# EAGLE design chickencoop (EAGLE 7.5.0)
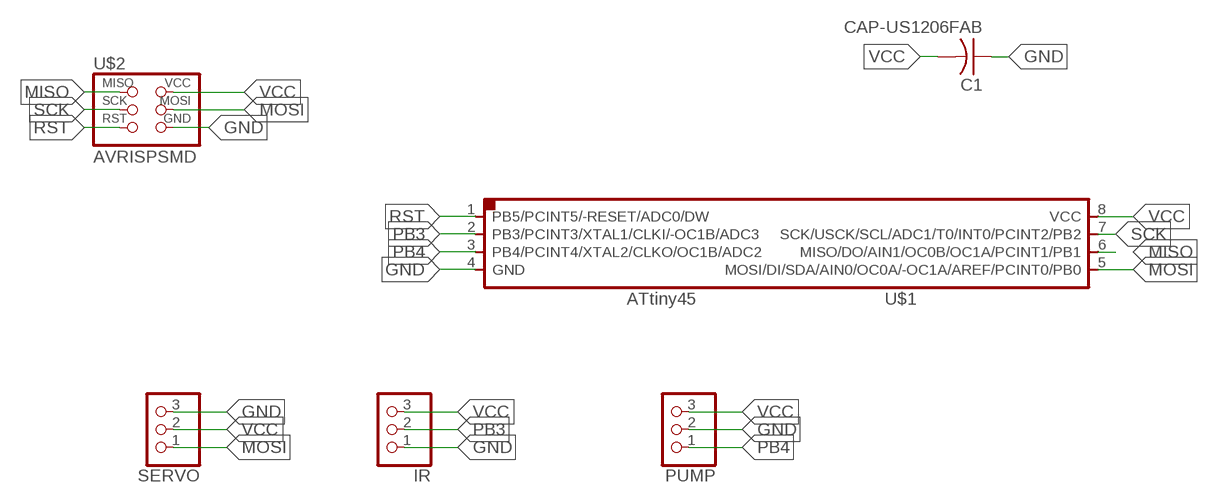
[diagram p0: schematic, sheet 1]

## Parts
C1  CAP-US1206FAB  [C1206FAB]
IR  PINHD-1X3  [1X03]
PUMP  PINHD-1X3  [1X03]
SERVO  PINHD-1X3  [1X03]
U$1  ATTINY45SI  [SOIC8]
U$2  AVRISPSMD  [2X03SMD]

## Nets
GND: C1.1 IR.1 PUMP.2 SERVO.3 U$1.4(GND) U$2.6(GND)
MISO: U$1.6(MISO/DO/AIN1/OC0B/OC1A/PCINT1/PB1) U$2.1(MISO)
MOSI: SERVO.1 U$1.5(MOSI/DI/SDA/AIN0/OC0A/-OC1A/AREF/PCINT0/PB0) U$2.4(MOSI)
PB3: IR.2 U$1.2(PB3/PCINT3/XTAL1/CLKI/-OC1B/ADC3)
PB4: PUMP.1 U$1.3(PB4/PCINT4/XTAL2/CLKO/OC1B/ADC2)
RST: U$1.1(PB5/PCINT5/-RESET/ADC0/DW) U$2.5(RST)
SCK: U$1.7(SCK/USCK/SCL/ADC1/T0/INT0/PCINT2/PB2) U$2.3(SCK)
VCC: C1.2 IR.3 PUMP.3 SERVO.2 U$1.8(VCC) U$2.2(VCC)

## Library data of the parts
C1 = fab:CAP-US
IR PUMP SERVO = pinhead:PINHD-1X3: PIN HEADER
U$1 = fab:ATTINY45
U$2 = fab:AVRISP

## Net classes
0 default: width 0.406 mm, drill 0.406 mm, clearance 0.406 mm

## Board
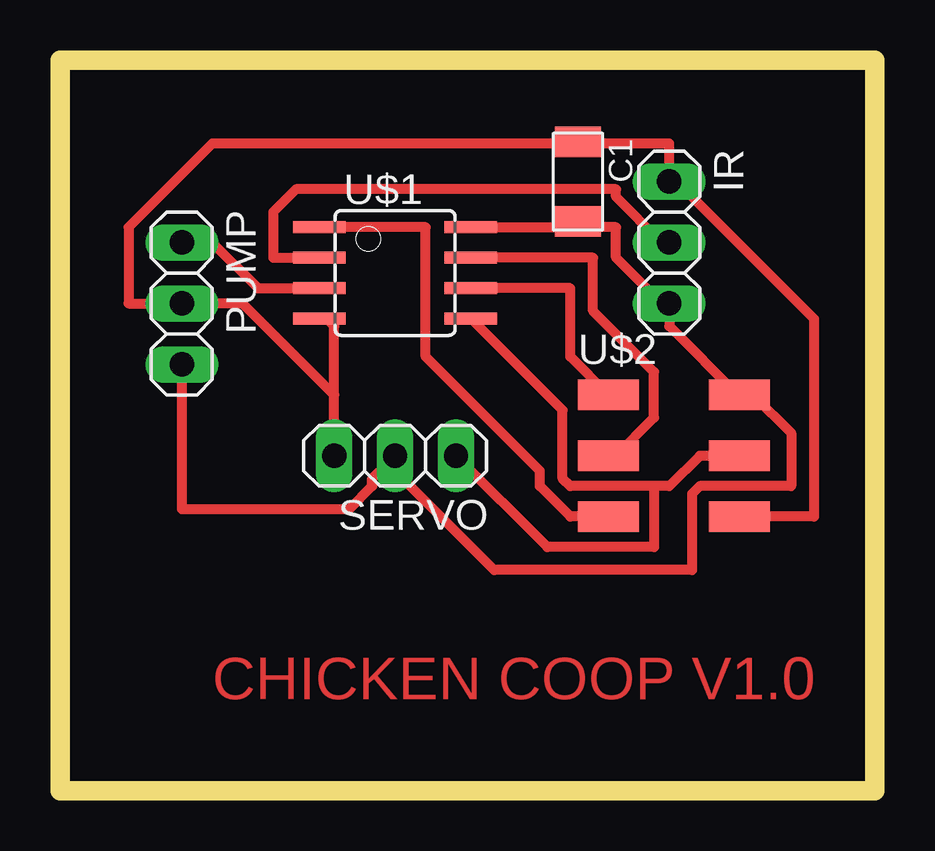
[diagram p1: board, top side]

Size 33.96 x 30.47 mm. Coordinates in mm from the lower left corner, seen from the top.
Outline: 0,0 33.96,0 33.96,30.47 0,30.47 0,0
Copper layers (1*16): Top 0.035mm / dielectric 1.5mm / Bottom 0.035mm
Design rules "default *": minimum track width 10mil, minimum drill 24mil, track to track 17mil, track to pad 17mil, pad to pad 17mil, via to via 17mil, smd to smd 8mil, copper to edge 40mil, drill to drill 8mil, minimum pad ring 10mil, minimum via ring 8mil, stop-mask expansion 4mil, vias tented up to drill 0mil, thermal gap 10mil

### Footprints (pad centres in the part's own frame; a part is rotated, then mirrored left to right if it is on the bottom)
C1206FAB = smd 1.27 x 1.905: 1 -1.651,0; 2 1.651,0
1X03 = drill 1.016 long: 1 -2.54,0; 2 0,0; 3 2.54,0
SOIC8 = smd 0.5 x 2.2: 1 -1.905,-3.154; 2 -0.645,-3.154; 3 0.625,-3.154; 4 1.895,-3.154; 5 1.905,3.154; 6 0.635,3.154; 7 -0.635,3.154; 8 -1.905,3.154
2X03SMD = smd 2.54 x 1.27: 1 -2.54,2.54; 2 2.92,2.54; 3 -2.54,0; 4 2.92,0; 5 -2.54,-2.54; 6 2.92,-2.54

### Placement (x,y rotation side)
C1  21.59,25.4 270 top
IR  25.4,22.86 270 top
PUMP  5.08,20.32 270 top
SERVO  13.97,13.97 180 top
U$1  13.97,21.59 270 top
U$2  25.4,13.97 0 top

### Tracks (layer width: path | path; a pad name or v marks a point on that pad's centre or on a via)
GND
  Top 0.406: SERVO.3 11.43,16.51 | 11.43,16.51 11.43,19.37 11.11,19.69 U$1.4 | 11.43,16.51 7.62,20.32 PUMP.2 2.86,20.32 2.86,23.49 6.35,26.99 21.59,26.99 | 21.59,26.99 25.4,26.99 25.4,25.72 | U$2.6 31.43,11.43 31.43,19.69 25.4,25.72 | 25.4,25.72 IR.1 | 21.59,26.99 C1.1
MISO
  Top 0.406: U$1.6 21.27,20.95 21.27,18.1 U$2.1
MOSI
  Top 0.406: 24.76,12.7 25.4,12.7 26.67,13.97 U$2.4 | 24.76,12.7 21.27,12.7 20.95,13.02 20.95,15.88 17.14,19.69 U$1.5 | SERVO.1 20.32,10.16 24.76,10.16 24.76,12.7
PB3
  Top 0.406: IR.2 25.08,22.86 23.18,24.77 23.18,25.08 9.84,25.08 8.89,24.13 8.89,22.23 10.79,22.23 U$1.2
PB4
  Top 0.406: PUMP.1 6.35,22.86 8.25,20.95 10.79,20.95 U$1.3
RST
  Top 0.406: U$1.1 15.24,23.49 15.24,18.1 20,13.34 20,12.7 21.27,11.43 U$2.5
SCK
  Top 0.406: U$1.7 22.22,22.23 22.22,20 24.76,17.46 24.76,15.56 23.18,13.97 U$2.3
VCC
  Top 0.406: 13.65,13.65 13.02,13.02 13.02,12.7 12.06,11.75 5.08,11.75 PUMP.3 | U$1.8 21.59,23.49 | 25.4,20 25.4,19.37 28.26,16.51 U$2.2 28.89,16.51 30.48,14.92 30.48,12.7 26.67,12.7 26.35,12.38 26.35,9.21 18.1,9.21 13.65,13.65 | 21.59,23.49 23.18,23.49 23.18,22.23 25.4,20 | 21.59,23.49 C1.2 | 25.4,20 IR.3 | 13.65,13.65 SERVO.2

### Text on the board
Top: CHICKEN COOP V1.0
